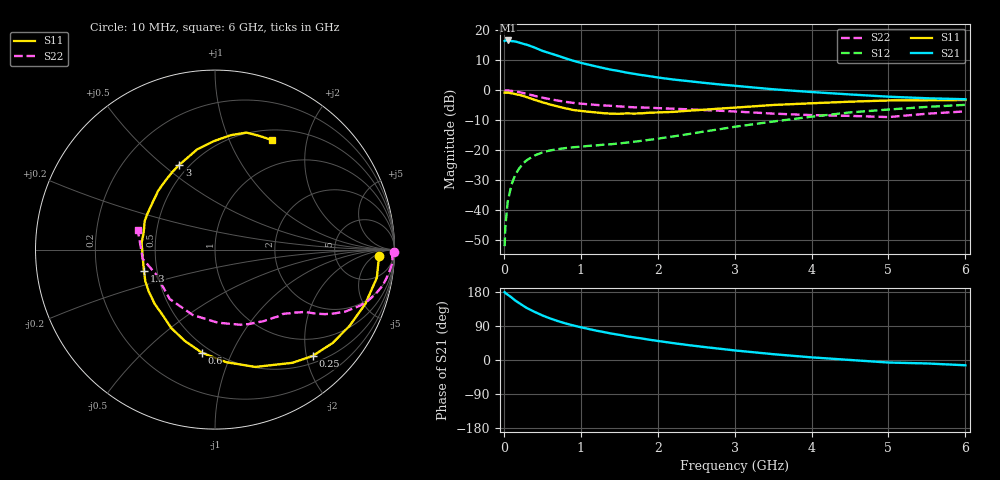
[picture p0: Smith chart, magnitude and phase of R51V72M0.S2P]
! SIEMENS Small Signal Semiconductors
! BFR183
! Si NPN RF Bipolar Junction Transistor in SOT23
! VCE = 1.75 V  IC = 2 mA
! Common Emitter S-Parameters:  May  1996
# GHz  S  MA  R  50
!  f  S11  S21  S12  S22
! GHz  MAG  ANG  MAG  ANG  MAG  ANG  MAG  ANG
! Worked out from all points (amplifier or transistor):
!   36 points, 10 MHz to 6 GHz, reference 50 ohm
!   highest |S21| = 16.6 dB at 50 MHz (marker M1)
!   |S21| within 3 dB of that: start of sweep to 458 MHz
!   unconditionally stable (mu >= 1): 1.373 GHz to 2.88 GHz
!   at 250 MHz: K = 0.23, MSG = 20.0 dB, |S12| = -24.4 dB
!   at 1.4 GHz: K = 1.01, MAG = 11.7 dB, |S12| = -18.0 dB
!   at 6 GHz: K = 0.92, MSG = 0.9 dB, |S12| = -4.9 dB
!   S11 on the Smith chart (normalised r, x): 10 MHz: 19, -8; 250 MHz: 0.63, -2.12; 600 MHz: 0.45, -0.77; 1.3 GHz: 0.42, -0.12; 3 GHz: 0.44, +0.57; 6 GHz: 0.63, +1.46
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0.01  0.915 -2.1  6.646 178.9  0.0025 89.4  0.9963 -0.8
0.02  0.9133 -4.2  6.756 176.8  0.0054 90.7  0.9869 -1.5
0.05  0.9152 -9.9  6.775 172.4  0.0137 85.1  0.9918 -4.2
0.1  0.8902 -19.9  6.607 165.1  0.0268 79.6  0.9754 -8.1
0.15  0.8619 -29.5  6.51 156.8  0.039 73.4  0.9564 -12.0
0.25  0.8046 -47.4  5.967 143.5  0.06 64.5  0.9003 -18.3
0.3  0.7644 -55.6  5.739 137.1  0.0683 60.7  0.8687 -21.0
0.4  0.6914 -71.0  5.157 127.1  0.0816 54.3  0.8059 -25.3
0.5  0.6305 -84.3  4.551 117.7  0.0916 49.5  0.7532 -28.2
0.6  0.5788 -97.3  4.142 109.8  0.0989 46.0  0.7103 -30.4
0.7  0.5354 -108.4  3.774 102.8  0.1041 43.9  0.6728 -32.1
0.8  0.5005 -119.1  3.416 96.7  0.1083 42.2  0.6407 -33.4
0.9  0.4685 -128.1  3.11 91.3  0.1117 41.6  0.6151 -34.5
1.1  0.4376 -147.2  2.676 82.0  0.1178 40.9  0.5832 -36.9
1.3  0.4134 -163.1  2.337 73.7  0.1236 42.0  0.5577 -39.0
1.6  0.4109 174.7  1.966 62.5  0.1339 45.1  0.5278 -42.6
2.2  0.4354 143.1  1.512 44.6  0.1696 51.2  0.4918 -52.2
3  0.5124 112.9  1.189 25.3  0.2455 51.8  0.4423 -71.2
3.5  0.5676 100.0  1.038 15.4  0.3002 48.1  0.4075 -87.8
4.5  0.6441 82.0  0.851 0.1  0.4267 36.2  0.3734 -132.5
5.5  0.6809 67.8  0.735 -9.1  0.5274 21.6  0.4059 -172.6
6  0.6877 62.5  0.708 -13.9  0.571 12.5  0.4438 165.7
